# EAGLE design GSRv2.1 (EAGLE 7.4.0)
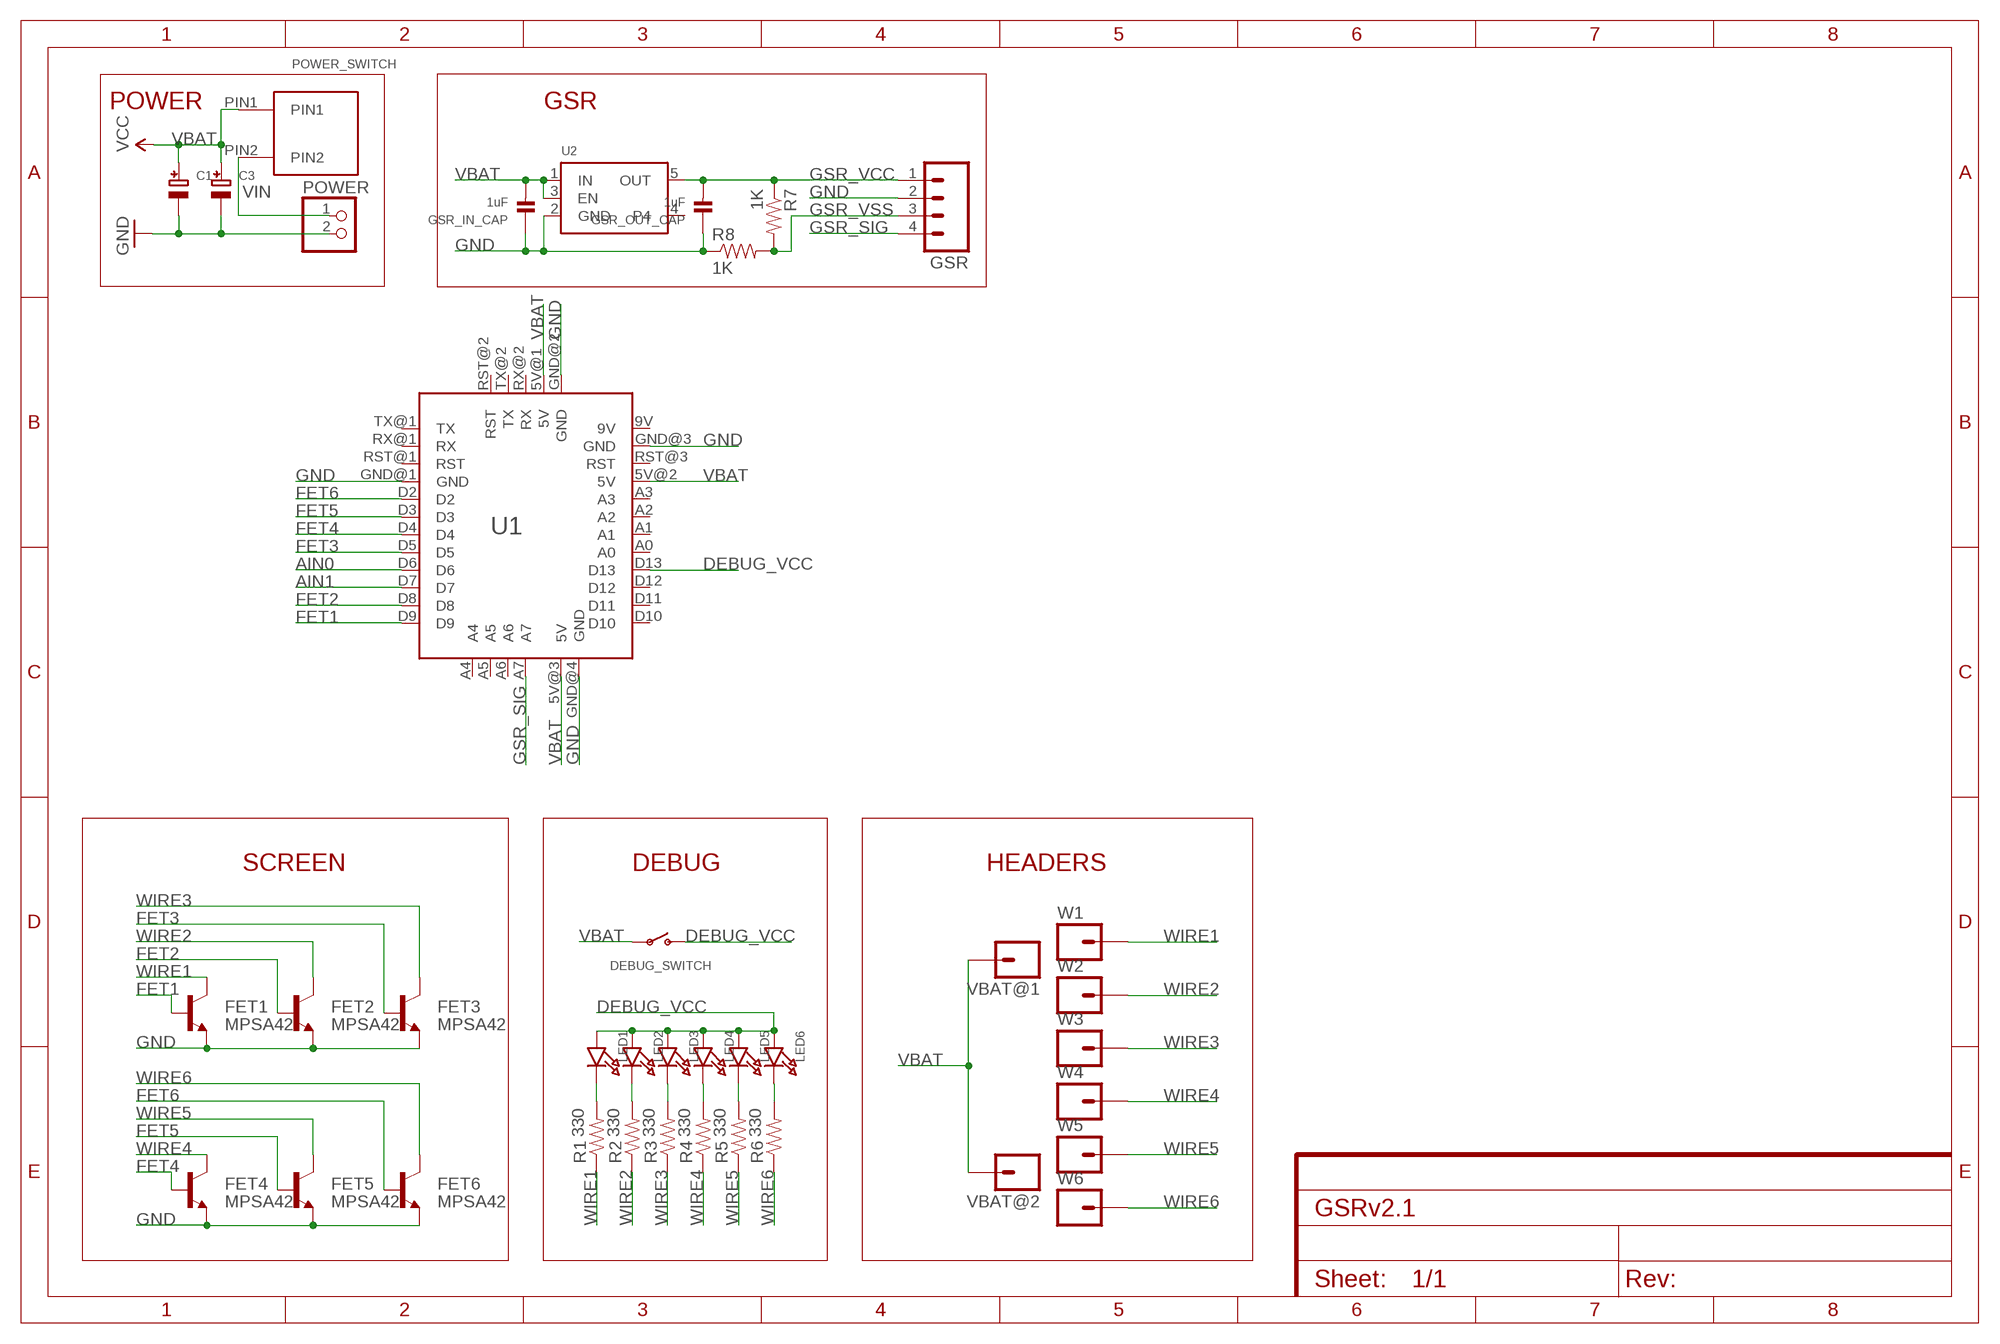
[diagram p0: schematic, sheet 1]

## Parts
C1  CAP_TANTALUMB/3528_WAVE  [EIA3528-21/B-W]
C3  CAP_TANTALUMB/3528_WAVE  [EIA3528-21/B-W]
DEBUG_SWITCH  SWITCH_SPST  [SPST_SMT_19192]
FET1  MPSA42  TRANSISTOR_NPNMPSA42  [SOT23-3]
FET2  MPSA42  TRANSISTOR_NPNMPSA42  [SOT23-3]
FET3  MPSA42  TRANSISTOR_NPNMPSA42  [SOT23-3]
FET4  MPSA42  TRANSISTOR_NPNMPSA42  [SOT23-3]
FET5  MPSA42  TRANSISTOR_NPNMPSA42  [SOT23-3]
FET6  MPSA42  TRANSISTOR_NPNMPSA42  [SOT23-3]
GSR  M04PTH  [1X04]
GSR_IN_CAP  1uF  CAP_CERAMIC0603  [0603]
GSR_OUT_CAP  1uF  CAP_CERAMIC0603  [0603]
LED1  LED0603_NOOUTLINE  [CHIPLED_0603_NOOUTLINE]
LED2  LED0603_NOOUTLINE  [CHIPLED_0603_NOOUTLINE]
LED3  LED0603_NOOUTLINE  [CHIPLED_0603_NOOUTLINE]
LED4  LED0603_NOOUTLINE  [CHIPLED_0603_NOOUTLINE]
LED5  LED0603_NOOUTLINE  [CHIPLED_0603_NOOUTLINE]
LED6  LED0603_NOOUTLINE  [CHIPLED_0603_NOOUTLINE]
POWER  JST_2PIN  [JSTPH2]
POWER_SWITCH  PUSH_BUTTON  [PUSH_BUTTON]
R1  330  RESISTOR0603-RES  [0603-RES]
R2  330  RESISTOR0603-RES  [0603-RES]
R3  330  RESISTOR0603-RES  [0603-RES]
R4  330  RESISTOR0603-RES  [0603-RES]
R5  330  RESISTOR0603-RES  [0603-RES]
R6  330  RESISTOR0603-RES  [0603-RES]
R7  1K  0OHM-1/10W-5%(0603)  [0603]
R8  1K  0OHM-1/10W-5%(0603)  [0603]
U1  ARDUINO_MINI  [ARDUINO_MINI]
U2  VREG_SOT23-5  [SOT23-5]
VBAT@1  M01NOSILK-KIT  [1X01NS-KIT]
VBAT@2  M01NOSILK-KIT  [1X01NS-KIT]
W1  M01NOSILK-KIT  [1X01NS-KIT]
W2  M01NOSILK-KIT  [1X01NS-KIT]
W3  M01NOSILK-KIT  [1X01NS-KIT]
W4  M01NOSILK-KIT  [1X01NS-KIT]
W5  M01NOSILK-KIT  [1X01NS-KIT]
W6  M01NOSILK-KIT  [1X01NS-KIT]

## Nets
AIN0: U1.D6
AIN1: U1.D7
DEBUG_VCC: DEBUG_SWITCH.C(S) LED1.A LED2.A LED3.A LED4.A LED5.A LED6.A U1.D13
FET1: FET1.1(B) U1.D9
FET2: FET2.1(B) U1.D8
FET3: FET3.1(B) U1.D5
FET4: FET4.1(B) U1.D4
FET5: FET5.1(B) U1.D3
FET6: FET6.1(B) U1.D2
GND: C1.- C3.- FET1.2(E) FET2.2(E) FET3.2(E) FET4.2(E) FET5.2(E) FET6.2(E) GSR.2 GSR_IN_CAP.1 GSR_OUT_CAP.1 POWER.2 R8.1 U1.GND@1(GND) U1.GND@2(GND) U1.GND@3(GND) U1.GND@4(GND) U2.2(GND)
GSR_SIG: GSR.4 U1.A7
GSR_VCC: GSR.1 GSR_OUT_CAP.2 R7.1 U2.5(OUT)
GSR_VSS: GSR.3 R7.2 R8.2
N$1: LED1.C R1.2
N$2: LED2.C R2.2
N$3: LED3.C R3.2
N$4: LED4.C R4.2
N$5: LED5.C R5.2
N$6: LED6.C R6.2
VBAT: C1.+ C3.+ DEBUG_SWITCH.B(P) GSR_IN_CAP.2 POWER_SWITCH.PIN1 U1.5V@1(5V) U1.5V@2(5V) U1.5V@3(5V) U2.1(IN) U2.3(EN) VBAT@1.1 VBAT@2.1 ; supply symbol labelled VCC
VIN: POWER.1 POWER_SWITCH.PIN2
WIRE1: FET1.3(C) R1.1 W1.1
WIRE2: FET2.3(C) R2.1 W2.1
WIRE3: FET3.3(C) R3.1 W3.1
WIRE4: FET4.3(C) R4.1 W4.1
WIRE5: FET5.3(C) R5.1 W5.1
WIRE6: FET6.3(C) R6.1 W6.1
Unconnected: U1.A0 U1.A1 U1.A2 U1.A3 U1.A4 U1.A5 U1.A6 U1.D10 U1.D11 U1.D12 U1.RST@1(RST) U1.RST@2(RST) U1.RST@3(RST) U1.RX@1(RX) U1.RX@2(RX) U1.TX@1(TX) U1.TX@2(TX) U2.4

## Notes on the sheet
- POWER | GSR
- SCREEN | DEBUG | HEADERS

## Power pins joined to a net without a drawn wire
9V: U1.9V

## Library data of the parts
C1 C3 = microbuilder:CAP_TANTALUM: Tantalum Capacitors
DEBUG_SWITCH = microbuilder:SWITCH_SPST: Switch - SPST
FET1-FET6 = SparkFun-DiscreteSemi:TRANSISTOR_NPN: Generic NPN BJT MMBT2222A - TRANS-08049 (SOT-23, 1A 40V) MPSA42 - TRANS-09116 (SOT-23, 500mA 300V) MMBT5088LT1G - TRANS-11160 (SOT-23, 50 mA 30V) BC547 - COM-08928 (TO-92 45V 100mA) (1.Collector 2.Base 3.Emitter) 2N3904 - COM-00521 (TO-92 40V 200mA) (1.Emitter 2.Base 3.Collector) P2N2222A -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; PROD_ID: TRANS-09116
GSR = SparkFun-Connectors:M04: Header 4 Standard 4-pin 0.1" header. Use with straight break away headers (SKU : PRT-00116), right angle break away headers (PRT-00553), swiss pins (PRT-00743), machine pins (PRT-00117), and female headers (PRT-00115). Molex polarized connector foot print use with SKU : PRT-08231 with associated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
GSR_IN_CAP GSR_OUT_CAP = microbuilder:CAP_CERAMIC: Ceramic Capacitors
LED1-LED6 = microbuilder:LED: LED
POWER = microbuilder:JST_2PIN: JST 2-Pin Right-Angle Connector
POWER_SWITCH = myParts:PUSH_BUTTON
R1-R6 = SparkFun-Passives:RESISTOR: Resistor
R7 R8 = SparkFun-Resistors:0OHM-1/10W-5%(0603): RES-08609; PROD_ID: RES-08609; VALUE: 0
U1 = myParts:ARDUINO_MINI: Arduino Mini V5 Footprint
U2 = microbuilder:VREG_SOT23-5: SOT23-5 Fixed Voltage Regulators To better organise some of the SOT23-5 fixed voltage regulators in this library, this new part was created. Part Current Out V Out V In V Dropout Digikey Part No. ADP121 150mA 3.3V 3.4-5.5V 0.09V @ 150mA ADP121-AUJZ33R7CT-ND ADP121 150mA 3.0V 3.1-5.5V 0.09V @ 150mA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
VBAT@1 VBAT@2 W1-W6 = SparkFun-Connectors:M01: Header 1

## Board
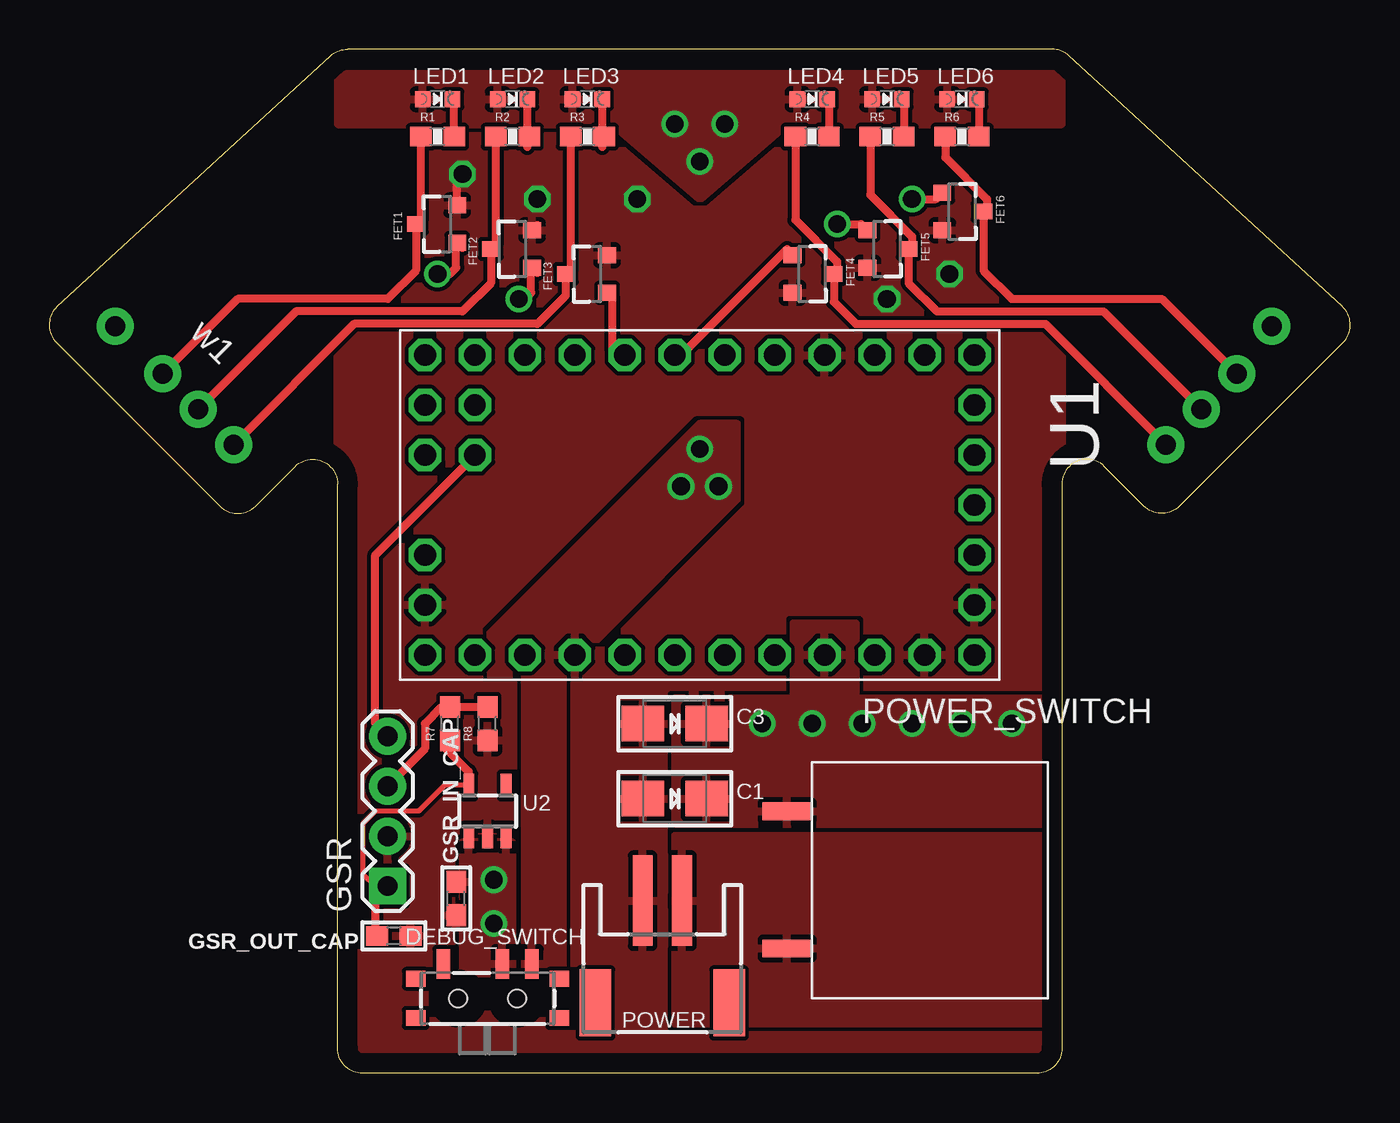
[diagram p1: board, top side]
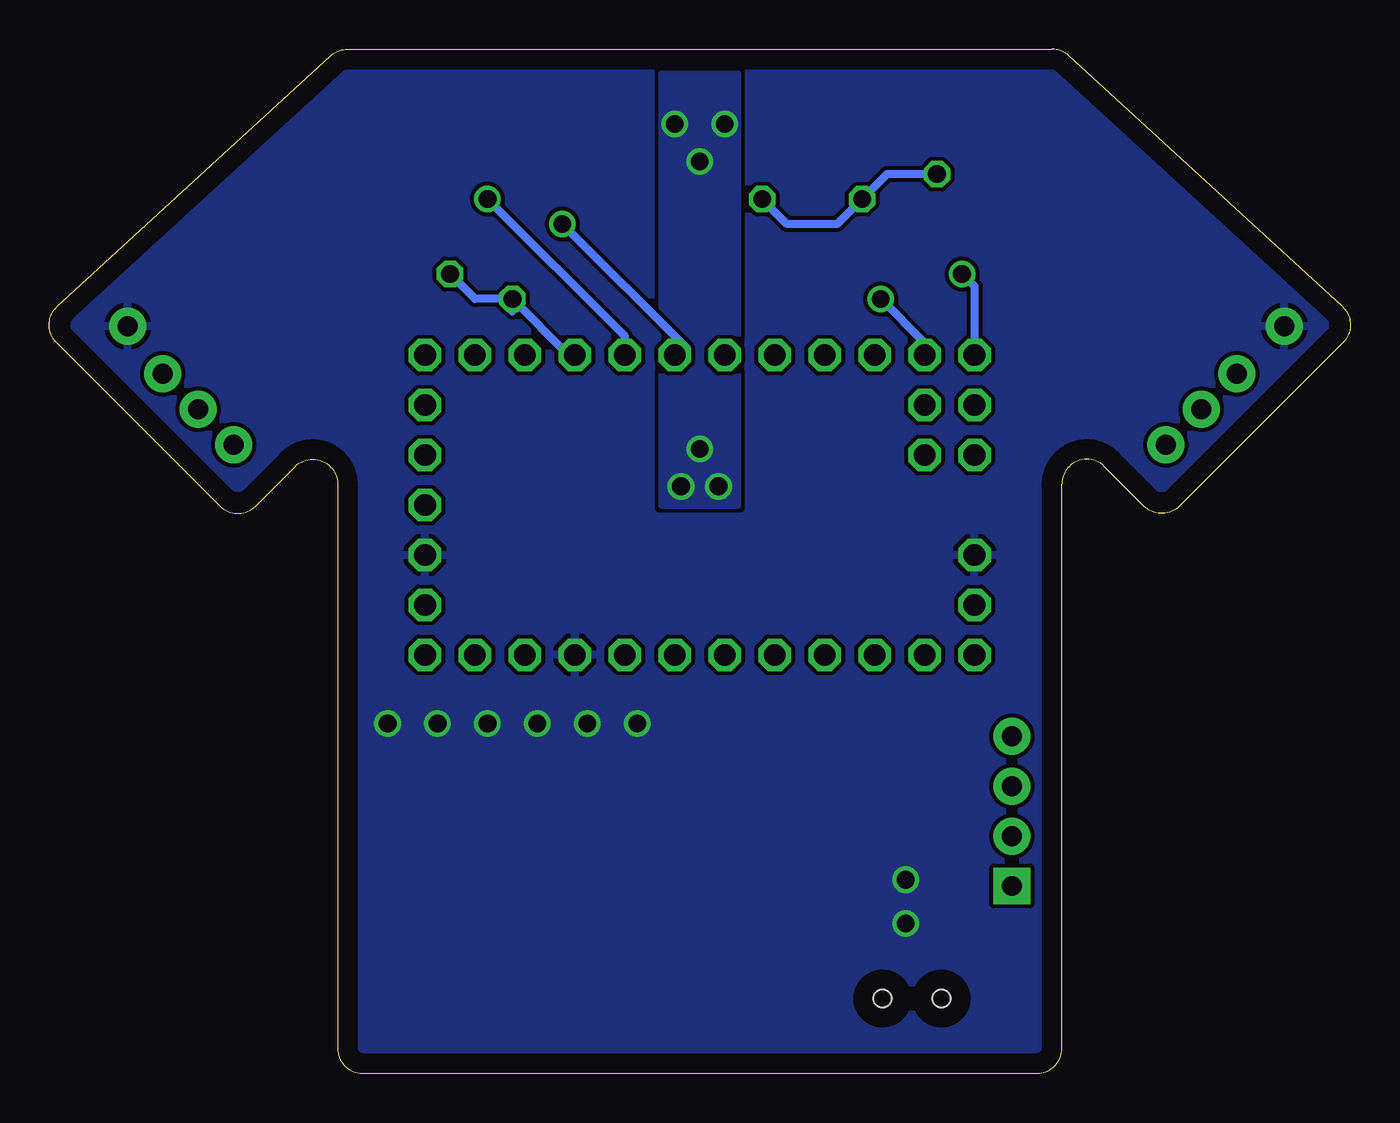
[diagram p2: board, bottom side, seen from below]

Size 66.18 x 52.07 mm. Coordinates in mm from the lower left corner, seen from the top.
Outline: 0.41,39 14.31,51.74 arc-43 15.17,52.07 51.01,52.07 arc-43 51.87,51.74 65.77,39 arc-92 65.81,37.16 57.48,28.84 arc-90 55.69,28.84 53.67,30.85 arc135 51.5,29.95 51.5,1.27 arc-90 50.23,0 15.94,0 arc-90 14.67,1.27 14.67,29.95 arc135 12.51,30.85 10.49,28.84 arc-90 8.7,28.84 0.37,37.16 arc-92 0.41,39
Copper layers (1*16): Top 0.035mm / dielectric 1.5mm / Bottom 0.035mm
Design rules "default": minimum track width 10mil, minimum drill 24mil, track to track 8mil, track to pad 8mil, pad to pad 8mil, via to via 8mil, smd to smd 8mil, copper to edge 40mil, drill to drill 8mil, minimum pad ring 10mil, minimum via ring 8mil, stop-mask expansion 4mil, vias tented up to drill 0mil, thermal gap 10mil

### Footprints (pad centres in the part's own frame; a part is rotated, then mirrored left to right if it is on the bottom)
EIA3528-21/B-W = smd 2.15 x 1.8: + 1.625,0; - -1.625,0
SPST_SMT_19192 = smd 0.7 x 1.5: A -2.25,1.75; B 0.75,1.75; C 2.25,1.75 | smd 1 x 0.8: GND1 -3.65,1; GND2 -3.65,-1; GND3 3.65,1; GND4 3.65,-1 | hole 0.9: -1.5,0; 1.5,0
SOT23-3 = smd 0.8 x 0.9: 1 -0.95,-1; 2 0.95,-1; 3 0,1.1
1X04 = drill 1.016 pad 1.88 square: 1 0,0 | drill 1.016 pad 1.88: 2 2.54,0; 3 5.08,0; 4 7.62,0
0603 = smd 1.1 x 1: 1 -0.85,0; 2 0.85,0
CHIPLED_0603_NOOUTLINE = smd 0.8 x 0.8: A 0,-0.75; C 0,0.75
JSTPH2 = smd 1 x 4.6: 1 -1,-3.7; 2 1,-3.7 | smd 1.6 x 3.4: NC1 -3.4,1.5; NC2 3.4,1.5
PUSH_BUTTON = smd 2.5 x 0.9: PIN1 -13.97,-0.644; PIN2 -13.97,-7.62
0603-RES = smd 1.1 x 1: 1 -0.85,0; 2 0.85,0
ARDUINO_MINI = drill 1.1 octagon: 5V@1 2.54,15.24; 5V@2 7.62,7.62; 5V@3 2.54,-12.7; 9V 7.62,15.24; A0 7.62,-2.54; A1 7.62,0; A2 7.62,2.54; A3 7.62,5.08; A4 -5.08,-12.7; A5 -2.54,-12.7; A6 -5.08,-10.16; A7 -2.54,-10.16; D2 -7.62,5.08; D3 -7.62,2.54; D4 -7.62,0; D5 -7.62,-2.54; D6 -7.62,-5.08; D7 -7.62,-7.62; D8 -7.62,-10.16; D9 -7.62,-12.7; D10 7.62,-12.7; D11 7.62,-10.16; D12 7.62,-7.62; D13 7.62,-5.08; GND@1 -7.62,7.62; GND@2 5.08,15.24; GND@3 7.62,12.7; GND@4 5.08,-12.7; RST@1 -7.62,10.16; RST@2 -5.08,15.24; RST@3 7.62,10.16; RX@1 -7.62,12.7; RX@2 0,15.24; TX@1 -7.62,15.24; TX@2 -2.54,15.24
SOT23-5 = smd 0.55 x 1.2: 1 -0.95,-1.3; 2 0,-1.3; 3 0.95,-1.3; 4 0.95,1.3; 5 -0.95,1.3
1X01NS-KIT = drill 1.016 pad 1.88: 1 0,0

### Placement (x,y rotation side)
C1  31.82,13.97 0 top
C3  31.82,17.78 0 top
DEBUG_SWITCH  22.29,3.81 0 top
FET1  19.75,43.18 90 top
FET2  23.56,41.91 90 top
FET3  27.37,40.64 90 top
FET4  38.8,40.64 270 top
FET5  42.61,41.91 270 top
FET6  46.42,43.81 270 top
GSR  17.21,9.53 90 top
GSR_IN_CAP  20.71,8.89 90 top
GSR_OUT_CAP  17.53,6.99 180 top
LED1  19.75,49.53 270 top
LED2  23.56,49.53 270 top
LED3  27.37,49.53 270 top
LED4  38.8,49.53 270 top
LED5  42.61,49.53 270 top
LED6  46.42,49.53 270 top
POWER  31.18,5.08 180 top
POWER_SWITCH  51.5,13.97 0 top
R1  19.75,47.62 0 top
R2  23.56,47.62 0 top
R3  27.37,47.62 0 top
R4  38.8,47.62 0 top
R5  42.61,47.62 0 top
R6  46.42,47.62 0 top
R7  20.39,17.78 90 top
R8  22.29,17.78 90 top
U1  31.82,28.89 270 top
U2  22.29,13.34 0 top
VBAT@1  3.35,37.99 135 top
VBAT@2  62.19,37.99 315 top
W1  5.78,35.56 45 top
W2  7.58,33.76 45 top
W3  9.38,31.97 45 top
W4  56.8,31.97 315 top
W5  58.6,33.76 315 top
W6  60.39,35.56 315 top

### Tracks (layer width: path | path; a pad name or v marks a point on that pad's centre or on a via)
DEBUG_VCC  (via drill 0.9)
  other vias: 33.09,31.75 32.14,29.84 34.04,29.84 33.09,46.35 31.82,48.26 34.36,48.26
  pour Bottom: 34.99,28.89 34.99,50.8 31.18,50.8 31.18,28.89
  pour Top: 33.09,44.45 37.53,48.26 51.5,48.26 51.5,50.8 14.67,50.8 14.67,48.26 28.64,48.26
  pour Top: 20.39,20.32 27.37,20.32 27.37,21.59 34.99,29.21 34.99,33.02 33.09,33.02
  pour Top: 24.2,5.08 24.2,21.59 26.1,21.59 26.1,5.08
FET1  (via drill 0.9)
  Top 0.406: 21.02,41.96 FET1.1 20.71,42.18 20.71,40.96 20.39,40.64 v19.75,40.64
  Bottom 0.406: v19.75,40.64 19.12,40.01 U1.D9
FET2  (via drill 0.9)
  Top 0.406: 24.83,40.69 FET2.1 24.52,40.91 24.52,39.69 24.2,39.37 v23.88,39.37
  Bottom 0.406: U1.D8 21.66,37.15 v23.88,39.37
FET3
  Top 0.406: U1.D5 28.96,36.51 28.64,36.83 28.64,39.42 FET3.1
FET4
  Top 0.406: 37.8,41.55 FET4.1 37.53,41.86 37.53,41.91 32.14,36.51 U1.D4
FET5  (via drill 0.9)
  Top 0.406: v40.07,43.18 41.29,43.18 FET5.1
  Bottom 0.406: U1.D3 33.72,36.83 v40.07,43.18
FET6  (via drill 0.9)
  Top 0.406: v43.88,44.45 45.1,44.45 FET6.1
  Bottom 0.406: U1.D2 36.9,37.46 v43.88,44.45
GND  (via drill 0.9)
  Top 0.406: FET1.2 20.75,45.45 v21.02,45.72 | FET2.2 24.83,43.13
  Bottom 0.406: v42.61,39.37 42.61,38.73 | v21.02,45.72 23.56,45.72 v24.83,44.45 26.1,43.18 28.64,43.18 v29.91,44.45 | U1.GND@1 39.76,36.51 v42.61,39.37 | 45.15,40.01 v45.79,40.64 44.52,39.37 v42.61,39.37
  pour Top (rank 3): 14.67,58.42 51.5,58.42 51.5,-6.35 14.67,-6.35
GSR_SIG
  Top 0.406: GSR.4 16.58,17.78 16.58,26.35 U1.A7
GSR_VCC
  Top 0.254: U2.5 20.1,14.64 18.8,13.34 16.58,13.34 15.94,12.7 15.94,10.16 16.58,9.53 GSR.1
  Top 0.406: R7.1 20.07,16.61 21.34,15.34 U2.5 | 16.58,9.53 16.58,7.09 GSR_OUT_CAP.2
GSR_VSS
  Top 0.406: R8.2 R7.2 19.97,18.63 19.12,17.78 19.12,16.51 GSR.3
N$1
  Top 0.406: R1.2 20.6,49.43 LED1.C
N$2
  Top 0.406: LED2.C 24.31,47.09 R2.2
N$3
  Top 0.406: LED3.C 28.12,47.09 R3.2
N$4
  Top 0.406: LED4.C 39.65,49.43 R4.2
N$5
  Top 0.406: LED5.C 43.46,49.43 R5.2
N$6
  Top 0.406: LED6.C 47.27,49.43 R6.2
VBAT  (via drill 0.9)
  other vias: 22.61,9.84 22.61,7.62 41.34,17.78 38.8,17.78 36.26,17.78 43.88,17.78 46.42,17.78 48.96,17.78
  pour Bottom (rank 2): -6.92,55.88 76.9,54.61 76.9,-3.81 -6.92,-2.54
  pour Top: 51.5,19.05 41.03,19.05 41.03,22.86 37.85,22.86 37.85,19.05 31.82,19.05 31.82,12.7 51.5,12.7
  pour Top: 23.56,11.75 21.02,11.75 21.02,5.08 23.56,5.08
VIN
  pour Top: 51.5,12.07 31.82,12.07 31.82,2.54 51.5,2.54
WIRE1
  Top 0.406: W1.1 9.59,39.37 17.21,39.37 18.65,40.81 FET1.3 18.9,43.43 R1.1
WIRE2
  Top 0.406: W2.1 12.55,38.73 21.02,38.73 22.46,40.17 FET2.3 22.71,42.16 R2.1
WIRE3
  Top 0.406: W3.1 15.51,38.1 24.83,38.1 26.27,39.54 FET3.3 26.52,40.89 R3.1
WIRE4
  Top 0.406: W4.1 50.67,38.1 41.03,38.1 39.9,39.22 FET4.3 40.07,40.81 40.07,41.27 37.95,43.39 R4.1
WIRE5
  Top 0.406: W5.1 53.63,38.73 45.15,38.73 43.71,40.17 FET5.3 43.88,42.08 43.88,42.55 41.76,44.66 R5.1
WIRE6
  Top 0.406: W6.1 56.58,39.37 48.96,39.37 47.52,40.81 FET6.3 47.69,43.98 47.69,44.45 45.57,46.57 R6.1

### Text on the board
tSilk: w1

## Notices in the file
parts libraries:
SparkFun-Aesthetics: Licensing: Creative Commons ShareAlike 4.0 International - https://creativecommons.org/licenses/by-sa/4.0
microbuilder: This work is placed in the public domain, and may be freely used for commercial and non-commercial work with the following conditions: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
